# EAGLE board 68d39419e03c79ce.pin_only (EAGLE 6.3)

Size 21.59 x 27.94 mm. Coordinates in mm from the lower left corner, seen from the top.
Outline: 2.54,27.94 19.05,27.94 arc-90 21.59,25.4 21.59,2.54 arc-90 19.05,0 2.54,0 arc-90 0,2.54 0,25.4 arc-90 2.54,27.94
Copper layers (1*16): Top 0.035mm / dielectric 1.5mm / Bottom 0.035mm
Design rules "adafruit": minimum track width 8mil, minimum drill 15.5mil, track to track 8mil, track to pad 8mil, pad to pad 8mil, via to via 8mil, smd to smd 8mil, copper to edge 10mil, drill to drill 8mil, minimum pad ring 10mil, minimum via ring 8mil, stop-mask expansion 4mil, vias tented up to drill 20mil, thermal gap 10mil

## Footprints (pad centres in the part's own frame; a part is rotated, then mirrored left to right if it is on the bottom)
0805-NO = smd 1.3 x 1.5: 1 -0.95,0; 2 0.95,0
_0805MP = smd 1.2 x 1.3: 1 -1.016,0; 2 1.016,0
FIDUCIAL_1MM = smd 1 x 1: 1 0,0
QFN20_4MM = smd 0.73 x 0.28: P$1 -1.965,1; P$2 -1.965,0.5; P$3 -1.965,0; P$4 -1.965,-0.5; P$5 -1.965,-1; P$11 1.965,-1; P$12 1.965,-0.5; P$13 1.965,0; P$14 1.965,0.5; P$15 1.965,1 | smd 0.28 x 0.73: P$6 -1,-1.965; P$7 -0.5,-1.965; P$8 0,-1.965; P$9 0.5,-1.965; P$10 1,-1.965; P$16 1,1.965; P$17 0.5,1.965; P$18 0,1.965; P$19 -0.5,1.965; P$20 -1,1.965 | smd 2.5 x 2.5: P$21 0,0
TERMBLOCK_1X2-3.5MM = drill 1 pad 2.184: 1 1.8,0; 2 -1.7,0
1X10_ROUND70 = drill 1 pad 1.778 square: 1 -11.43,0 | drill 1 pad 1.778: 2 -8.89,0; 3 -6.35,0; 4 -3.81,0; 5 -1.27,0; 6 1.27,0; 7 3.81,0; 8 6.35,0; 9 8.89,0; 10 11.43,0
MOUNTINGHOLE_2.5_PLATED_THICK = drill 2.5 pad 4: P$1 0,0

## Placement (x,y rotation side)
C1  10µF  [0805-NO]  6.05,24.21 270 top
C2  0.1µF  [0805-NO]  11.32,18.62 90 top
C3  0.1µF  [0805-NO]  12.98,23.36 180 top
C4  0.1µF  [0805-NO]  9.11,25.18 180 top
C5  1µF  [0805-NO]  6.03,10.19 0 top
C6  1µF  [0805-NO]  6.03,12.36 0 top
C7  1µF  [0805-NO]  6.03,15.87 0 top
C8  1µF  [0805-NO]  6.03,17.81 0 top
C9  10µF  [0805-NO]  9.14,23.37 180 top
FB1  ferrite  [_0805MP]  12.98,25.18 0 top
FB2  ferrite  [_0805MP]  10.76,21.59 0 top
FID1  FIDUCIAL""  [FIDUCIAL_1MM]  3.49,27 0 top
FID2  FIDUCIAL""  [FIDUCIAL_1MM]  15.67,1.3 0 top
FID3  FIDUCIAL""  [FIDUCIAL_1MM]  13.46,9.02 0 top
IC1  TPA2016D2QFN  [QFN20_4MM]  11.3,13.84 90 top
J1  [TERMBLOCK_1X2-3.5MM]  18.03,10.16 90 top
J2  [TERMBLOCK_1X2-3.5MM]  18.03,17.78 90 top
JP1  [1X10_ROUND70]  1.52,13.97 270 top
R1  10K  [0805-NO]  7.07,7.34 0 top
R2  10K  [0805-NO]  7.09,4.98 0 top
R3  100K  [0805-NO]  6.99,20.57 90 top
U$3  [ADAFRUIT_5MM]  9.4,4.45 0 top
U$4  [ADAFRUIT_3.5MM]  11.81,14.61 0 bottom
U$20  MOUNTINGHOLE2.5_THICK  [MOUNTINGHOLE_2.5_PLATED_THICK]  19.05,2.54 0 top
U$21  MOUNTINGHOLE2.5_THICK  [MOUNTINGHOLE_2.5_PLATED_THICK]  19.05,25.4 0 top

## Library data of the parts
C1-C9 FB1 FB2 IC1 J1 J2 JP1 R1-R3 U$3 U$4 = microbuilder
FID1-FID3 U$20 U$21 = microbuilder; BOM: EXCLUDE

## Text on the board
tPlace: TPA2016D2 | VDD | GND | RIGHT | + | SHDN | R- | R+ | - | L+ | L- | SCL | SDA | LEFT | + | Class D Stereo / Audio Amp | I2C / Vcc
bPlace: TPA2016D2 / Class D / Stereo Amp / w/AGC & I2C / Volume Ctrl | VDD & I2C Vcc: / 2.5-5.5VDC | Max Output / Pwr @ 5V: | (per speaker) | 2.8W @ 4Ohm | 1.7W @ 8Ohm | 6dB Default Gain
